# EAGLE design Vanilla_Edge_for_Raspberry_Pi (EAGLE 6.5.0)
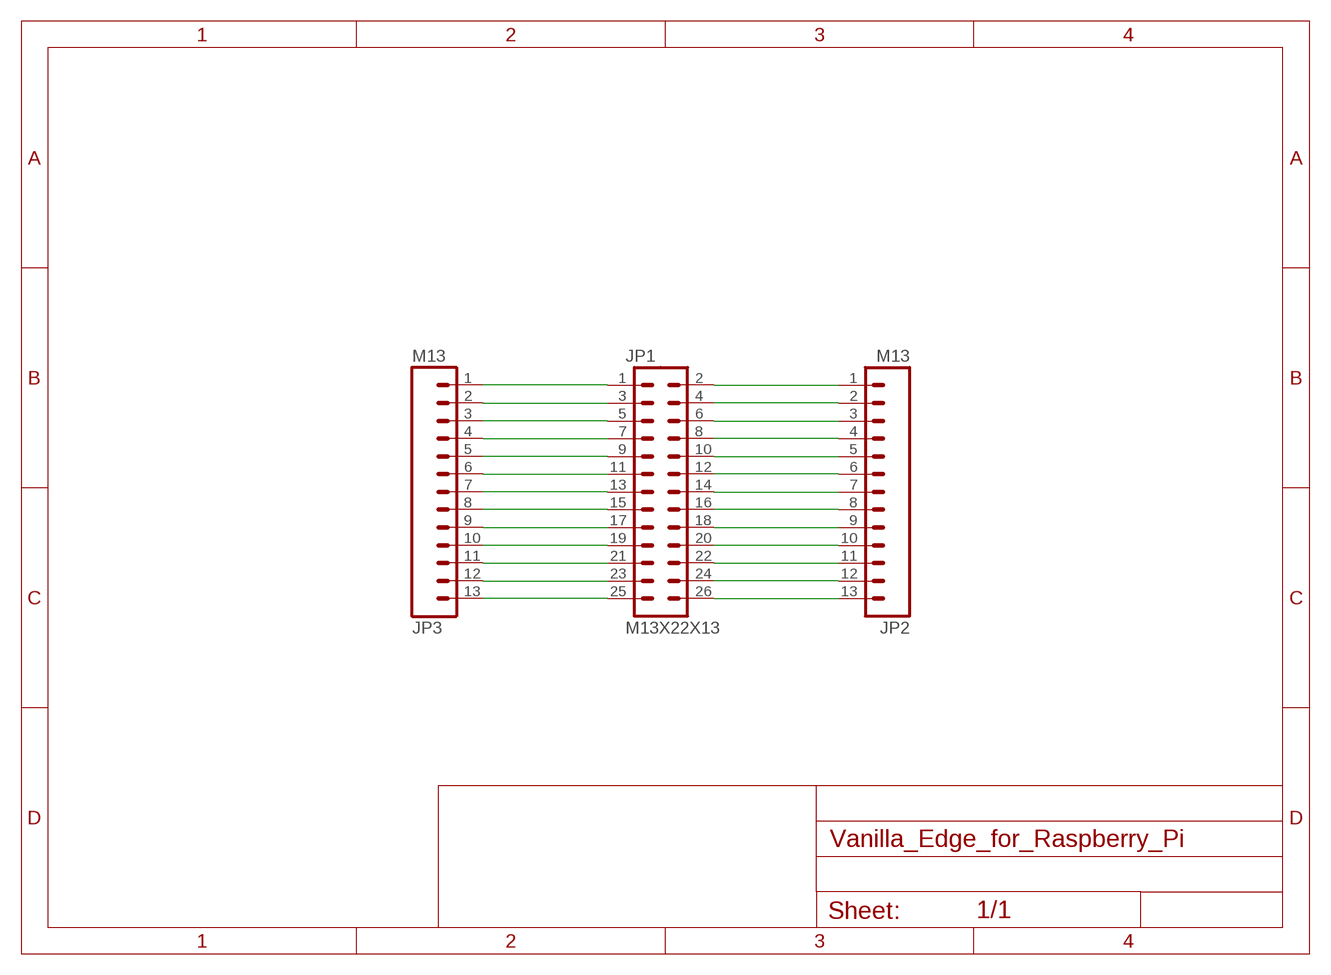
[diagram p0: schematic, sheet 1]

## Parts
JP1  M13X22X13  [2X13]
JP2  M13  [M13]
JP3  M13  [M13]

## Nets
N$1: JP1.1 JP3.1
N$2: JP1.3 JP3.2
N$3: JP1.5 JP3.3
N$4: JP1.7 JP3.4
N$5: JP1.9 JP3.5
N$6: JP1.11 JP3.6
N$7: JP1.13 JP3.7
N$8: JP1.15 JP3.8
N$9: JP1.17 JP3.9
N$10: JP1.19 JP3.10
N$11: JP1.21 JP3.11
N$12: JP1.23 JP3.12
N$13: JP1.25 JP3.13
N$14: JP1.26 JP2.13
N$15: JP1.24 JP2.12
N$16: JP1.22 JP2.11
N$17: JP1.20 JP2.10
N$18: JP1.18 JP2.9
N$19: JP1.16 JP2.8
N$20: JP1.14 JP2.7
N$21: JP1.12 JP2.6
N$22: JP1.10 JP2.5
N$23: JP1.8 JP2.4
N$24: JP1.6 JP2.3
N$25: JP1.4 JP2.2
N$26: JP1.2 JP2.1

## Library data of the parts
JP1 = SparkFun-Connectors:M13X2: 0.1" spaced headers
JP2 JP3 = M13:M13

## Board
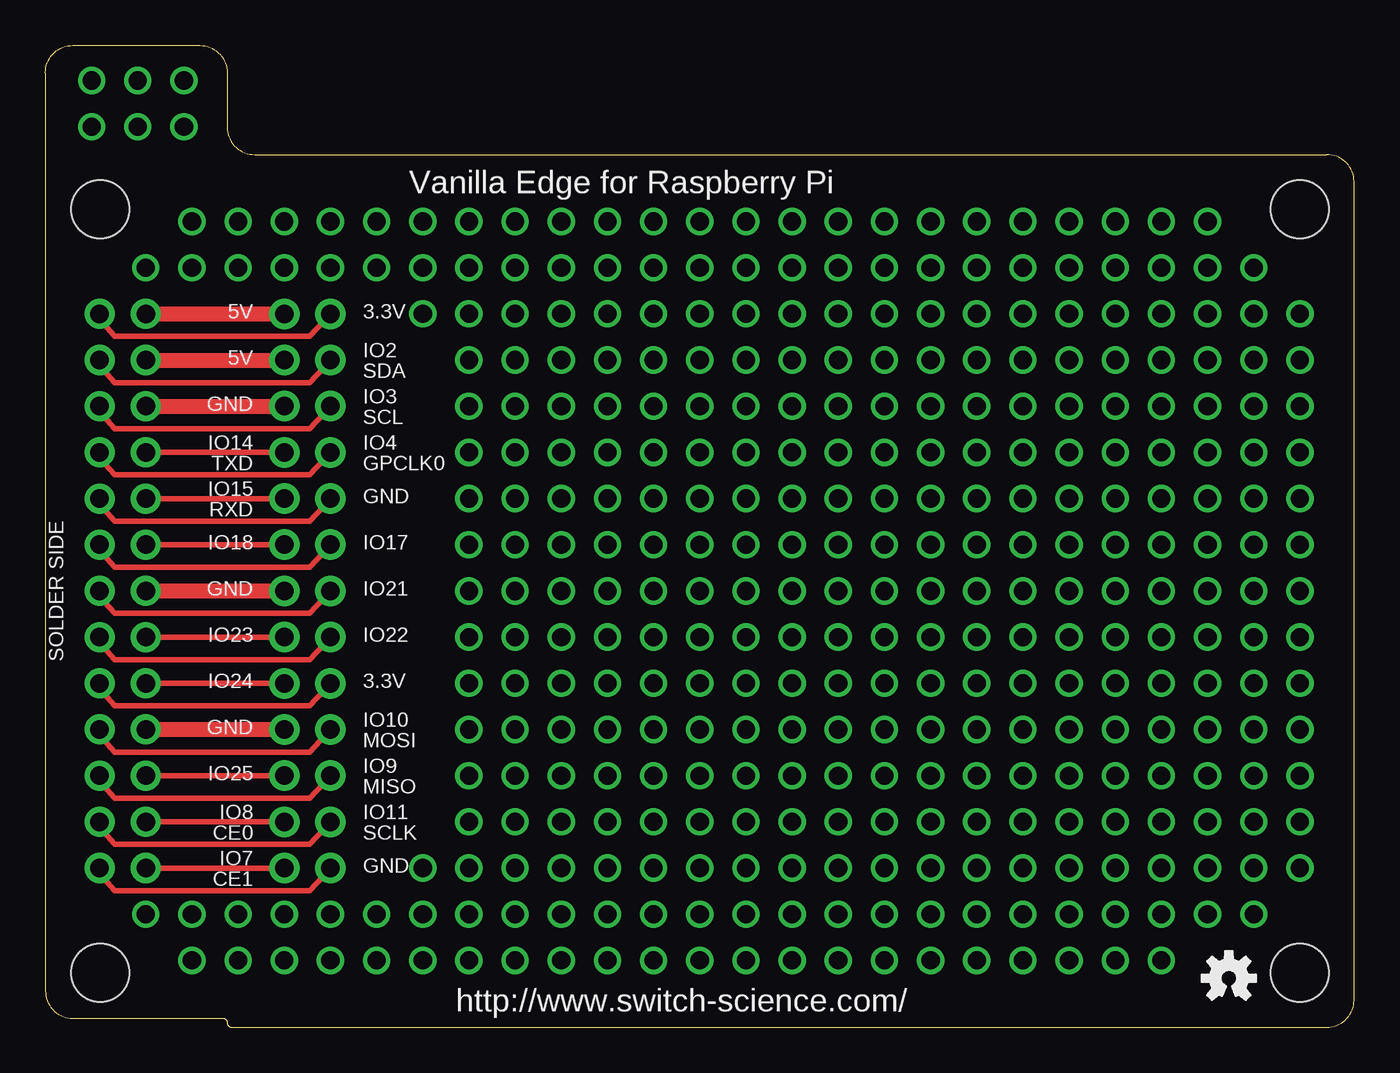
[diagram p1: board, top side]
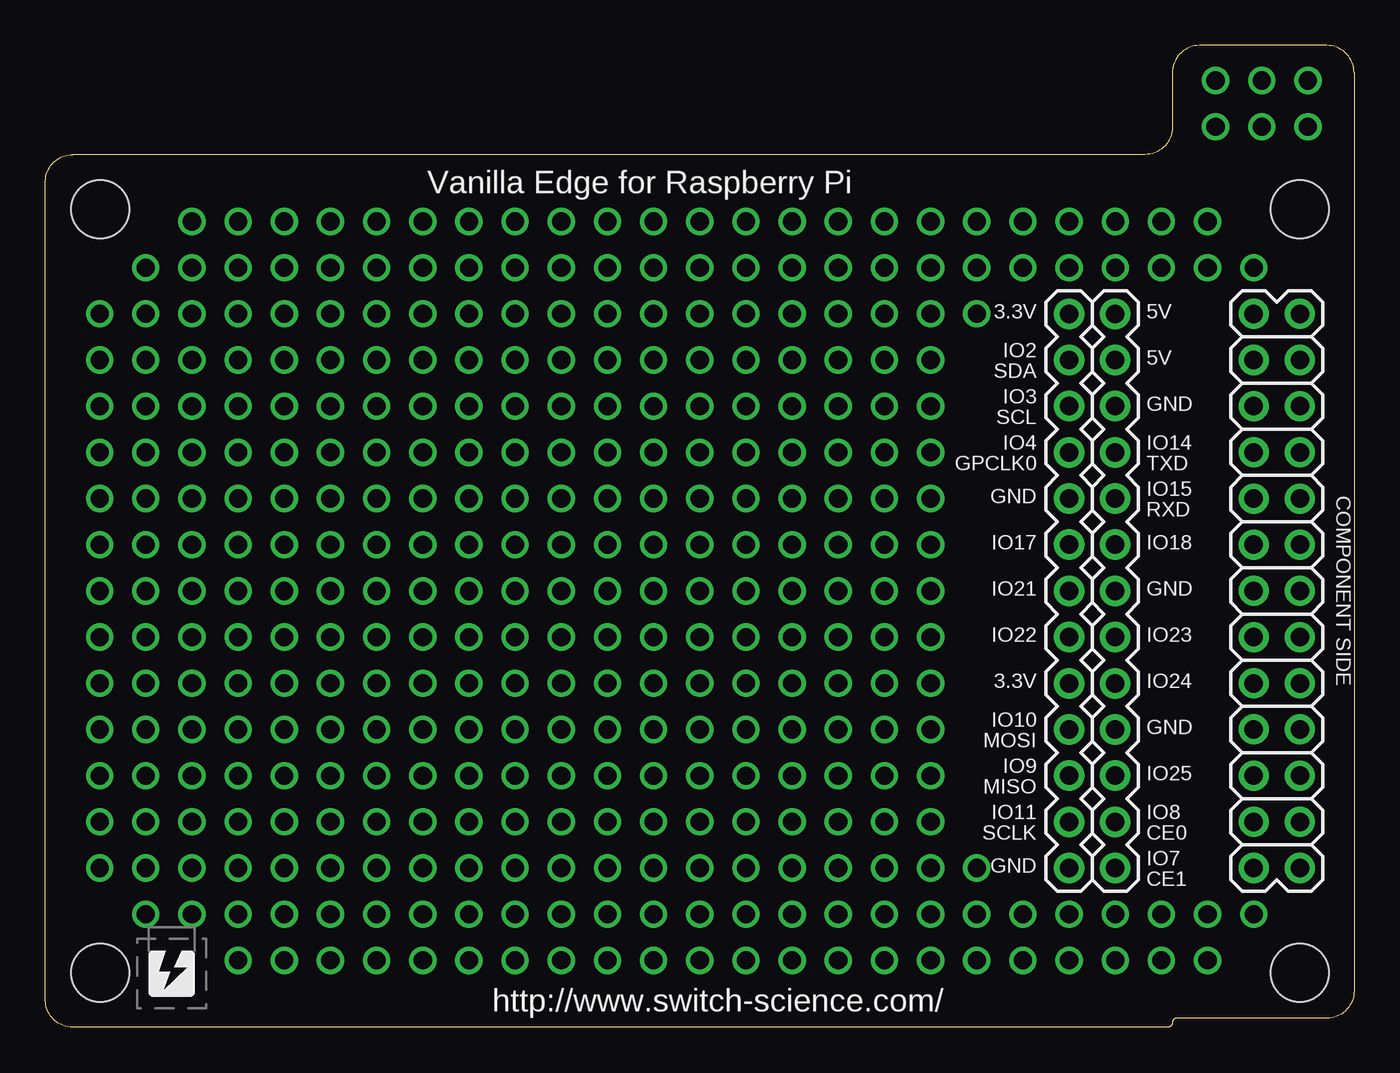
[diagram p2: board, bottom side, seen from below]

Size 72 x 54 mm. Coordinates in mm from the lower left corner, seen from the top.
Outline: 10,52.5 10,49.5 arc90 11.5,48 70.5,48 arc-90 72,46.5 72,1.5 arc-90 70.5,0 10.25,0 arc-90 10,0.25 arc90 9.75,0.5 1.5,0.5 arc-90 0,2 0,52.5 arc-90 1.5,54 8.5,54 arc-90 10,52.5
Copper layers (1*16): Top 0.035mm / dielectric 1.5mm / Bottom 0.035mm
Design rules "PCBCartFine": minimum track width 0.2mm, minimum drill 0.4mm, track to track 0.2mm, track to pad 0.2mm, pad to pad 0.2mm, via to via 0.2mm, smd to smd 0.2mm, copper to edge 0.2mm, drill to drill 0.2mm, minimum pad ring 0.1mm, minimum via ring 0.1mm, stop-mask expansion 4mil, vias tented up to drill 0.5mm, thermal gap 0.2mm
Holes 3.2 mm at 3,45 69,3 3,3 69,45

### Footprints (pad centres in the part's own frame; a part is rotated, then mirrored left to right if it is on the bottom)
2X13 = drill 1.016 pad 1.651: 1 0,0; 2 0,2.54; 3 2.54,0; 4 2.54,2.54; 5 5.08,0; 6 5.08,2.54; 7 7.62,0; 8 7.62,2.54; 9 10.16,0; 10 10.16,2.54; 11 12.7,0; 12 12.7,2.54; 13 15.24,0; 14 15.24,2.54; 15 17.78,0; 16 17.78,2.54; 17 20.32,0; 18 20.32,2.54; 19 22.86,0; 20 22.86,2.54; 21 25.4,0; 22 25.4,2.54; 23 27.94,0; 24 27.94,2.54; 25 30.48,0; 26 30.48,2.54
M13 = drill 1.016 pad 1.676: 1 0,0; 2 2.54,0; 3 5.08,0; 4 7.62,0; 5 10.16,0; 6 12.7,0; 7 15.24,0; 8 17.78,0; 9 20.32,0; 10 22.86,0; 11 25.4,0; 12 27.94,0; 13 30.48,0

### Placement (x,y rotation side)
JP1  2.98,8.76 90 bottom
JP2  13.14,8.76 90 bottom
JP3  15.68,8.76 90 bottom
U$1  [LOGO]  66.33,1.68 0 bottom
U$7  OSHW-LOGOS  [OSHW-LOGO-S]  65.11,2.69 0 top

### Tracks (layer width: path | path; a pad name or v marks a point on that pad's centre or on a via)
N$1
  Top 0.305: JP1.1 2.98,8.45 3.81,7.52 14.54,7.52 JP3.1
N$2
  Top 0.305: JP1.3 2.98,10.99 3.81,10.06 14.54,10.06 JP3.2
N$3
  Top 0.305: JP1.5 2.98,13.53 3.81,12.6 14.54,12.6 JP3.3
N$4
  Top 0.305: JP1.7 2.98,16.07 3.81,15.14 14.54,15.14 JP3.4
N$5
  Top 0.305: JP1.9 2.98,18.61 3.81,17.68 14.54,17.68 JP3.5
N$6
  Top 0.305: JP1.11 2.98,21.15 3.81,20.22 14.54,20.22 JP3.6
N$7
  Top 0.305: JP1.13 2.98,23.69 3.81,22.76 14.54,22.76 JP3.7
N$8
  Top 0.305: JP1.15 2.98,26.23 3.81,25.3 14.54,25.3 JP3.8
N$9
  Top 0.305: JP1.17 2.98,28.77 3.81,27.84 14.54,27.84 JP3.9
N$10
  Top 0.305: JP1.19 2.98,31.31 3.81,30.38 14.54,30.38 JP3.10
N$11
  Top 0.305: JP1.21 2.98,33.85 3.81,32.92 14.54,32.92 JP3.11
N$12
  Top 0.305: JP1.23 2.98,36.39 3.81,35.46 14.54,35.46 JP3.12
N$13
  Top 0.305: JP1.25 2.98,38.93 3.81,38 14.54,38 JP3.13
N$14
  Top 0.813: JP1.26 JP2.13
N$15
  Top 0.813: JP1.24 JP2.12
N$16
  Top 0.813: JP1.22 JP2.11
N$17
  Top 0.305: JP1.20 JP2.10
N$18
  Top 0.305: JP1.18 JP2.9
N$19
  Top 0.305: JP1.16 JP2.8
N$20
  Top 0.813: JP1.14 JP2.7
N$21
  Top 0.305: JP1.12 JP2.6
N$22
  Top 0.305: JP1.10 JP2.5
N$23
  Top 0.813: JP1.8 JP2.4
N$24
  Top 0.305: JP1.6 JP2.3
N$25
  Top 0.305: JP1.4 JP2.2
N$26
  Top 0.305: JP1.2 JP2.1
N$27  (via drill 1)
  other vias: 36,24
N$28  (via drill 1)
  other vias: 33.46,24
N$29  (via drill 1)
  other vias: 33.46,26.54
N$30  (via drill 1)
  other vias: 36,26.54
N$31  (via drill 1)
  other vias: 36,29.08
N$32  (via drill 1)
  other vias: 33.46,29.08
N$33  (via drill 1)
  other vias: 30.92,29.08
N$34  (via drill 1)
  other vias: 30.92,26.54
N$35  (via drill 1)
  other vias: 30.92,24
N$36  (via drill 1)
  other vias: 30.92,21.46
N$37  (via drill 1)
  other vias: 33.46,21.46
N$38  (via drill 1)
  other vias: 36,21.46
N$39  (via drill 1)
  other vias: 36,18.92
N$40  (via drill 1)
  other vias: 33.46,18.92
N$41  (via drill 1)
  other vias: 30.92,18.92
N$42  (via drill 1)
  other vias: 30.92,16.38
N$43  (via drill 1)
  other vias: 33.46,16.38
N$44  (via drill 1)
  other vias: 36,16.38
N$45  (via drill 1)
  other vias: 36,13.84
N$46  (via drill 1)
  other vias: 33.46,13.84
N$47  (via drill 1)
  other vias: 30.92,13.84
N$48  (via drill 1)
  other vias: 28.38,13.84
N$49  (via drill 1)
  other vias: 28.38,16.38
N$50  (via drill 1)
  other vias: 28.38,18.92
N$51  (via drill 1)
  other vias: 28.38,21.46
N$52  (via drill 1)
  other vias: 28.38,24
N$53  (via drill 1)
  other vias: 28.38,26.54
N$54  (via drill 1)
  other vias: 28.38,29.08
N$55  (via drill 1)
  other vias: 25.84,29.08
N$56  (via drill 1)
  other vias: 25.84,31.62
N$57  (via drill 1)
  other vias: 25.84,34.16
N$58  (via drill 1)
  other vias: 25.84,36.7
N$59  (via drill 1)
  other vias: 25.84,39.24
N$60  (via drill 1)
  other vias: 25.84,41.78
N$61  (via drill 1)
  other vias: 23.3,41.78
N$62  (via drill 1)
  other vias: 25.84,26.54
N$63  (via drill 1)
  other vias: 25.84,24
N$64  (via drill 1)
  other vias: 25.84,21.46
N$65  (via drill 1)
  other vias: 25.84,18.92
N$66  (via drill 1)
  other vias: 25.84,16.38
N$67  (via drill 1)
  other vias: 25.84,13.84
N$68  (via drill 1)
  other vias: 25.84,11.3
N$69  (via drill 1)
  other vias: 28.38,11.3
N$70  (via drill 1)
  other vias: 30.92,11.3
N$71  (via drill 1)
  other vias: 33.46,11.3
N$72  (via drill 1)
  other vias: 36,11.3
N$73  (via drill 1)
  other vias: 25.84,8.76
N$74  (via drill 1)
  other vias: 25.84,6.22
N$75  (via drill 1)
  other vias: 23.3,39.24
N$76  (via drill 1)
  other vias: 38.54,11.3
N$77  (via drill 1)
  other vias: 41.08,11.3
N$78  (via drill 1)
  other vias: 43.62,11.3
N$79  (via drill 1)
  other vias: 46.16,11.3
N$80  (via drill 1)
  other vias: 48.7,11.3
N$81  (via drill 1)
  other vias: 51.24,11.3
N$82  (via drill 1)
  other vias: 53.78,11.3
N$83  (via drill 1)
  other vias: 56.32,11.3
N$84  (via drill 1)
  other vias: 58.86,11.3
N$85  (via drill 1)
  other vias: 61.4,11.3
N$86  (via drill 1)
  other vias: 63.94,11.3
N$87  (via drill 1)
  other vias: 66.48,11.3
N$88  (via drill 1)
  other vias: 23.3,36.7
N$89  (via drill 1)
  other vias: 23.3,11.3
N$90  (via drill 1)
  other vias: 20.76,39.24
N$91  (via drill 1)
  other vias: 20.76,8.76
N$92  (via drill 1)
  other vias: 2.54,49.53
N$93  (via drill 1)
  other vias: 2.54,52.07
N$94  (via drill 1)
  other vias: 5.08,52.07
N$95  (via drill 1)
  other vias: 5.08,49.53
N$96  (via drill 1)
  other vias: 7.62,49.53
N$97  (via drill 1)
  other vias: 23.3,34.16
N$98  (via drill 1)
  other vias: 23.3,31.62
N$99  (via drill 1)
  other vias: 23.3,29.08
N$100  (via drill 1)
  other vias: 23.3,26.54
N$101  (via drill 1)
  other vias: 23.3,24
N$102  (via drill 1)
  other vias: 23.3,21.46
N$103  (via drill 1)
  other vias: 23.3,18.92
N$104  (via drill 1)
  other vias: 23.3,16.38
N$105  (via drill 1)
  other vias: 23.3,13.84
N$106  (via drill 1)
  other vias: 23.3,8.76
N$107  (via drill 1)
  other vias: 23.3,6.22
N$108  (via drill 1)
  other vias: 28.38,6.22
N$109  (via drill 1)
  other vias: 28.38,8.76
N$110  (via drill 1)
  other vias: 30.92,8.76
N$111  (via drill 1)
  other vias: 30.92,6.22
N$112  (via drill 1)
  other vias: 33.46,6.22
N$113  (via drill 1)
  other vias: 33.46,8.76
N$114  (via drill 1)
  other vias: 36,8.76
N$115  (via drill 1)
  other vias: 36,6.22
N$116  (via drill 1)
  other vias: 38.54,6.22
N$117  (via drill 1)
  other vias: 38.54,8.76
N$118  (via drill 1)
  other vias: 41.08,8.76
N$119  (via drill 1)
  other vias: 41.08,6.22
N$120  (via drill 1)
  other vias: 43.62,6.22
N$121  (via drill 1)
  other vias: 43.62,8.76
N$122  (via drill 1)
  other vias: 46.16,8.76
N$123  (via drill 1)
  other vias: 48.7,8.76
N$124  (via drill 1)
  other vias: 51.24,8.76
N$125  (via drill 1)
  other vias: 53.78,8.76
N$126  (via drill 1)
  other vias: 56.32,8.76
N$127  (via drill 1)
  other vias: 58.86,8.76
N$128  (via drill 1)
  other vias: 61.4,8.76
N$129  (via drill 1)
  other vias: 63.94,8.76
N$130  (via drill 1)
  other vias: 66.48,8.76
N$131  (via drill 1)
  other vias: 66.48,6.22
N$132  (via drill 1)
  other vias: 63.94,6.22
N$133  (via drill 1)
  other vias: 61.4,6.22
N$134  (via drill 1)
  other vias: 58.86,6.22
N$135  (via drill 1)
  other vias: 56.32,6.22
N$136  (via drill 1)
  other vias: 53.78,6.22
N$137  (via drill 1)
  other vias: 51.24,6.22
N$138  (via drill 1)
  other vias: 48.7,6.22
N$139  (via drill 1)
  other vias: 46.16,6.22
N$140  (via drill 1)
  other vias: 38.54,13.84
N$141  (via drill 1)
  other vias: 41.08,13.84
N$142  (via drill 1)
  other vias: 43.62,13.84
N$143  (via drill 1)
  other vias: 46.16,13.84
N$144  (via drill 1)
  other vias: 48.7,13.84
N$145  (via drill 1)
  other vias: 51.24,13.84
N$146  (via drill 1)
  other vias: 53.78,13.84
N$147  (via drill 1)
  other vias: 56.32,13.84
N$148  (via drill 1)
  other vias: 58.86,13.84
N$149  (via drill 1)
  other vias: 61.4,13.84
N$150  (via drill 1)
  other vias: 63.94,13.84
N$151  (via drill 1)
  other vias: 66.48,13.84
N$152  (via drill 1)
  other vias: 66.48,16.38
N$153  (via drill 1)
  other vias: 63.94,16.38
N$154  (via drill 1)
  other vias: 61.4,16.38
N$155  (via drill 1)
  other vias: 58.86,16.38
N$156  (via drill 1)
  other vias: 38.54,16.38
N$157  (via drill 1)
  other vias: 41.08,16.38
N$158  (via drill 1)
  other vias: 43.62,16.38
N$159  (via drill 1)
  other vias: 46.16,16.38
N$160  (via drill 1)
  other vias: 48.7,16.38
N$161  (via drill 1)
  other vias: 51.24,16.38
N$162  (via drill 1)
  other vias: 53.78,16.38
N$163  (via drill 1)
  other vias: 56.32,16.38
N$164  (via drill 1)
  other vias: 66.48,18.92
N$165  (via drill 1)
  other vias: 66.48,21.46
N$166  (via drill 1)
  other vias: 66.48,24
N$167  (via drill 1)
  other vias: 66.48,26.54
N$168  (via drill 1)
  other vias: 66.48,29.08
N$169  (via drill 1)
  other vias: 66.48,31.62
N$170  (via drill 1)
  other vias: 66.48,34.16
N$171  (via drill 1)
  other vias: 66.48,36.7
N$172  (via drill 1)
  other vias: 66.48,39.24
N$173  (via drill 1)
  other vias: 66.48,41.78
N$174  (via drill 1)
  other vias: 63.94,41.78
N$175  (via drill 1)
  other vias: 61.4,41.78
N$176  (via drill 1)
  other vias: 58.86,41.78
N$177  (via drill 1)
  other vias: 56.32,41.78
N$178  (via drill 1)
  other vias: 53.78,41.78
N$179  (via drill 1)
  other vias: 51.24,41.78
N$180  (via drill 1)
  other vias: 48.7,41.78
N$181  (via drill 1)
  other vias: 46.16,41.78
N$182  (via drill 1)
  other vias: 43.62,41.78
N$183  (via drill 1)
  other vias: 41.08,41.78
N$184  (via drill 1)
  other vias: 38.54,41.78
N$185  (via drill 1)
  other vias: 36,41.78
N$186  (via drill 1)
  other vias: 33.46,41.78
N$187  (via drill 1)
  other vias: 30.92,41.78
N$188  (via drill 1)
  other vias: 28.38,41.78
N$189  (via drill 1)
  other vias: 28.38,39.24
N$190  (via drill 1)
  other vias: 20.76,41.78
N$191  (via drill 1)
  other vias: 18.22,41.78
N$192  (via drill 1)
  other vias: 15.68,41.78
N$193  (via drill 1)
  other vias: 13.14,41.78
N$194  (via drill 1)
  other vias: 10.6,41.78
N$195  (via drill 1)
  other vias: 8.06,41.78
N$196  (via drill 1)
  other vias: 5.52,41.78
N$197  (via drill 1)
  other vias: 20.76,6.22
N$198  (via drill 1)
  other vias: 18.22,6.22
N$199  (via drill 1)
  other vias: 15.68,6.22
N$200  (via drill 1)
  other vias: 13.14,6.22
N$201  (via drill 1)
  other vias: 10.6,6.22
N$202  (via drill 1)
  other vias: 8.06,6.22
N$203  (via drill 1)
  other vias: 5.52,6.22
N$204  (via drill 1)
  other vias: 7.62,52.07
N$217  (via drill 1)
  other vias: 28.38,36.7
N$218  (via drill 1)
  other vias: 28.38,34.16
N$219  (via drill 1)
  other vias: 28.38,31.62
N$220  (via drill 1)
  other vias: 30.92,31.62
N$221  (via drill 1)
  other vias: 33.46,31.62
N$222  (via drill 1)
  other vias: 33.46,34.16
N$223  (via drill 1)
  other vias: 30.92,34.16
N$224  (via drill 1)
  other vias: 30.92,36.7
N$225  (via drill 1)
  other vias: 33.46,36.7
N$226  (via drill 1)
  other vias: 33.46,39.24
N$227  (via drill 1)
  other vias: 30.92,39.24
N$228  (via drill 1)
  other vias: 36,39.24
N$229  (via drill 1)
  other vias: 36,36.7
N$230  (via drill 1)
  other vias: 36,34.16
N$231  (via drill 1)
  other vias: 36,31.62
N$232  (via drill 1)
  other vias: 38.54,39.24
N$233  (via drill 1)
  other vias: 38.54,36.7
N$234  (via drill 1)
  other vias: 41.08,36.7
N$235  (via drill 1)
  other vias: 41.08,39.24
N$236  (via drill 1)
  other vias: 43.62,39.24
N$237  (via drill 1)
  other vias: 46.16,39.24
N$238  (via drill 1)
  other vias: 48.7,39.24
N$239  (via drill 1)
  other vias: 51.24,39.24
N$240  (via drill 1)
  other vias: 53.78,39.24
N$241  (via drill 1)
  other vias: 56.32,39.24
N$242  (via drill 1)
  other vias: 58.86,39.24
N$243  (via drill 1)
  other vias: 61.4,39.24
N$244  (via drill 1)
  other vias: 63.94,39.24
N$245  (via drill 1)
  other vias: 63.94,36.7
N$246  (via drill 1)
  other vias: 61.4,36.7
N$247  (via drill 1)
  other vias: 58.86,36.7
N$248  (via drill 1)
  other vias: 56.32,36.7
N$249  (via drill 1)
  other vias: 53.78,36.7
N$250  (via drill 1)
  other vias: 51.24,36.7
N$251  (via drill 1)
  other vias: 48.7,36.7
N$252  (via drill 1)
  other vias: 46.16,36.7
N$253  (via drill 1)
  other vias: 43.62,36.7
N$254  (via drill 1)
  other vias: 38.54,34.16
N$255  (via drill 1)
  other vias: 41.08,31.62
N$256  (via drill 1)
  other vias: 43.62,29.08
N$257  (via drill 1)
  other vias: 46.16,26.54
N$258  (via drill 1)
  other vias: 48.7,24
N$259  (via drill 1)
  other vias: 51.24,21.46
N$260  (via drill 1)
  other vias: 53.78,18.92
N$261  (via drill 1)
  other vias: 56.32,21.46
N$262  (via drill 1)
  other vias: 58.86,24
N$263  (via drill 1)
  other vias: 61.4,26.54
N$264  (via drill 1)
  other vias: 63.94,29.08
N$265  (via drill 1)
  other vias: 63.94,31.62
N$266  (via drill 1)
  other vias: 63.94,34.16
N$267  (via drill 1)
  other vias: 61.4,34.16
N$268  (via drill 1)
  other vias: 61.4,31.62
N$269  (via drill 1)
  other vias: 61.4,29.08
N$270  (via drill 1)
  other vias: 58.86,34.16
N$271  (via drill 1)
  other vias: 56.32,34.16
N$272  (via drill 1)
  other vias: 53.78,34.16
N$273  (via drill 1)
  other vias: 51.24,34.16
N$274  (via drill 1)
  other vias: 48.7,34.16
N$275  (via drill 1)
  other vias: 46.16,34.16
N$276  (via drill 1)
  other vias: 43.62,34.16
N$277  (via drill 1)
  other vias: 41.08,34.16
N$278  (via drill 1)
  other vias: 43.62,31.62
N$279  (via drill 1)
  other vias: 46.16,31.62
N$280  (via drill 1)
  other vias: 48.7,31.62
N$281  (via drill 1)
  other vias: 51.24,31.62
N$282  (via drill 1)
  other vias: 53.78,31.62
N$283  (via drill 1)
  other vias: 56.32,31.62
N$284  (via drill 1)
  other vias: 58.86,31.62
N$285  (via drill 1)
  other vias: 58.86,29.08
N$286  (via drill 1)
  other vias: 56.32,29.08
N$287  (via drill 1)
  other vias: 53.78,29.08
N$288  (via drill 1)
  other vias: 51.24,29.08
N$289  (via drill 1)
  other vias: 48.7,29.08
N$290  (via drill 1)
  other vias: 46.16,29.08
N$291  (via drill 1)
  other vias: 38.54,31.62
N$292  (via drill 1)
  other vias: 38.54,29.08
N$293  (via drill 1)
  other vias: 41.08,29.08
N$294  (via drill 1)
  other vias: 41.08,26.54
N$295  (via drill 1)
  other vias: 43.62,26.54
N$296  (via drill 1)
  other vias: 48.7,26.54
N$297  (via drill 1)
  other vias: 51.24,26.54
N$298  (via drill 1)
  other vias: 53.78,26.54
N$299  (via drill 1)
  other vias: 56.32,26.54
N$300  (via drill 1)
  other vias: 58.86,26.54
N$301  (via drill 1)
  other vias: 63.94,26.54
N$302  (via drill 1)
  other vias: 63.94,24
N$303  (via drill 1)
  other vias: 61.4,24
N$304  (via drill 1)
  other vias: 56.32,24
N$305  (via drill 1)
  other vias: 53.78,24
N$306  (via drill 1)
  other vias: 51.24,24
N$307  (via drill 1)
  other vias: 63.94,21.46
N$308  (via drill 1)
  other vias: 61.4,21.46
N$309  (via drill 1)
  other vias: 58.86,21.46
N$310  (via drill 1)
  other vias: 58.86,18.92
N$311  (via drill 1)
  other vias: 61.4,18.92
N$312  (via drill 1)
  other vias: 63.94,18.92
N$313  (via drill 1)
  other vias: 56.32,18.92
N$314  (via drill 1)
  other vias: 53.78,21.46
N$315  (via drill 1)
  other vias: 51.24,18.92
N$316  (via drill 1)
  other vias: 48.7,18.92
N$317  (via drill 1)
  other vias: 46.16,18.92
N$318  (via drill 1)
  other vias: 48.7,21.46
N$319  (via drill 1)
  other vias: 46.16,21.46
N$320  (via drill 1)
  other vias: 43.62,21.46
N$321  (via drill 1)
  other vias: 43.62,18.92
N$322  (via drill 1)
  other vias: 41.08,18.92
N$323  (via drill 1)
  other vias: 41.08,21.46
N$324  (via drill 1)
  other vias: 38.54,21.46
N$325  (via drill 1)
  other vias: 38.54,18.92
N$326  (via drill 1)
  other vias: 38.54,24
N$327  (via drill 1)
  other vias: 41.08,24
N$328  (via drill 1)
  other vias: 43.62,24
N$329  (via drill 1)
  other vias: 46.16,24
N$330  (via drill 1)
  other vias: 38.54,26.54
N$331  (via drill 1)
  other vias: 69.02,39.24
N$332  (via drill 1)
  other vias: 69.02,36.7
N$333  (via drill 1)
  other vias: 69.02,34.16
N$334  (via drill 1)
  other vias: 69.02,31.62
N$335  (via drill 1)
  other vias: 69.02,29.08
N$336  (via drill 1)
  other vias: 69.02,26.54
N$337  (via drill 1)
  other vias: 69.02,24
N$338  (via drill 1)
  other vias: 69.02,21.46
N$339  (via drill 1)
  other vias: 69.02,18.92
N$340  (via drill 1)
  other vias: 69.02,16.38
N$341  (via drill 1)
  other vias: 69.02,13.84
N$342  (via drill 1)
  other vias: 69.02,11.3
N$343  (via drill 1)
  other vias: 69.02,8.76
N$344  (via drill 1)
  other vias: 63.94,44.32
N$345  (via drill 1)
  other vias: 61.4,44.32
N$346  (via drill 1)
  other vias: 58.86,44.32
N$347  (via drill 1)
  other vias: 56.32,44.32
N$348  (via drill 1)
  other vias: 53.78,44.32
N$349  (via drill 1)
  other vias: 51.24,44.32
N$350  (via drill 1)
  other vias: 48.7,44.32
N$351  (via drill 1)
  other vias: 46.16,44.32
N$352  (via drill 1)
  other vias: 43.62,44.32
N$353  (via drill 1)
  other vias: 41.08,44.32
N$354  (via drill 1)
  other vias: 38.54,44.32
N$355  (via drill 1)
  other vias: 36,44.32
N$356  (via drill 1)
  other vias: 33.46,44.32
N$357  (via drill 1)
  other vias: 30.92,44.32
N$358  (via drill 1)
  other vias: 28.38,44.32
N$359  (via drill 1)
  other vias: 25.84,44.32
N$360  (via drill 1)
  other vias: 23.3,44.32
N$361  (via drill 1)
  other vias: 20.76,44.32
N$362  (via drill 1)
  other vias: 18.22,44.32
N$363  (via drill 1)
  other vias: 15.68,44.32
N$364  (via drill 1)
  other vias: 13.14,44.32
N$365  (via drill 1)
  other vias: 10.6,44.32
N$366  (via drill 1)
  other vias: 8.06,44.32
N$373  (via drill 1)
  other vias: 10.6,3.68
N$374  (via drill 1)
  other vias: 13.14,3.68
N$375  (via drill 1)
  other vias: 15.68,3.68
N$376  (via drill 1)
  other vias: 18.22,3.68
N$377  (via drill 1)
  other vias: 20.76,3.68
N$378  (via drill 1)
  other vias: 23.3,3.68
N$379  (via drill 1)
  other vias: 25.84,3.68
N$380  (via drill 1)
  other vias: 28.38,3.68
N$381  (via drill 1)
  other vias: 30.92,3.68
N$382  (via drill 1)
  other vias: 33.46,3.68
N$383  (via drill 1)
  other vias: 36,3.68
N$384  (via drill 1)
  other vias: 38.54,3.68
N$385  (via drill 1)
  other vias: 41.08,3.68
N$386  (via drill 1)
  other vias: 43.62,3.68
N$387  (via drill 1)
  other vias: 46.16,3.68
N$388  (via drill 1)
  other vias: 48.7,3.68
N$389  (via drill 1)
  other vias: 51.24,3.68
N$390  (via drill 1)
  other vias: 53.78,3.68
N$391  (via drill 1)
  other vias: 56.32,3.68
N$392  (via drill 1)
  other vias: 58.86,3.68
N$393  (via drill 1)
  other vias: 61.4,3.68
N$394  (via drill 1)
  other vias: 8.06,3.68

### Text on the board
tPlace: Vanilla Edge for Raspberry Pi | 5V | 3.3V | 5V | IO2 | SDA | GND | IO3 | SCL | IO14 | IO4 | TXD | GPCLK0 | IO15 | RXD | GND | IO18 | IO17 | SOLDER SIDE | GND | IO21 | IO23 | IO22 | IO24 | 3.3V | GND | IO10 | MOSI | IO25 | IO9 | MISO | CE0 | IO8 | IO11 | SCLK | CE1 | IO7 | GND | http://www.switch-science.com/
bPlace: Vanilla Edge for Raspberry Pi | 5V | 3.3V | 5V | IO2 | SDA | GND | IO3 | SCL | IO14 | IO4 | TXD | GPCLK0 | IO15 | RXD | GND | IO18 | IO17 | COMPONENT SIDE | GND | IO21 | IO23 | IO22 | IO24 | 3.3V | GND | IO10 | MOSI | IO25 | IO9 | MISO | CE0 | IO8 | IO11 | SCLK | CE1 | IO7 | GND | http://www.switch-science.com/
tDocu: 72x54mm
